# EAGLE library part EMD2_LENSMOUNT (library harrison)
EMD2 Chip
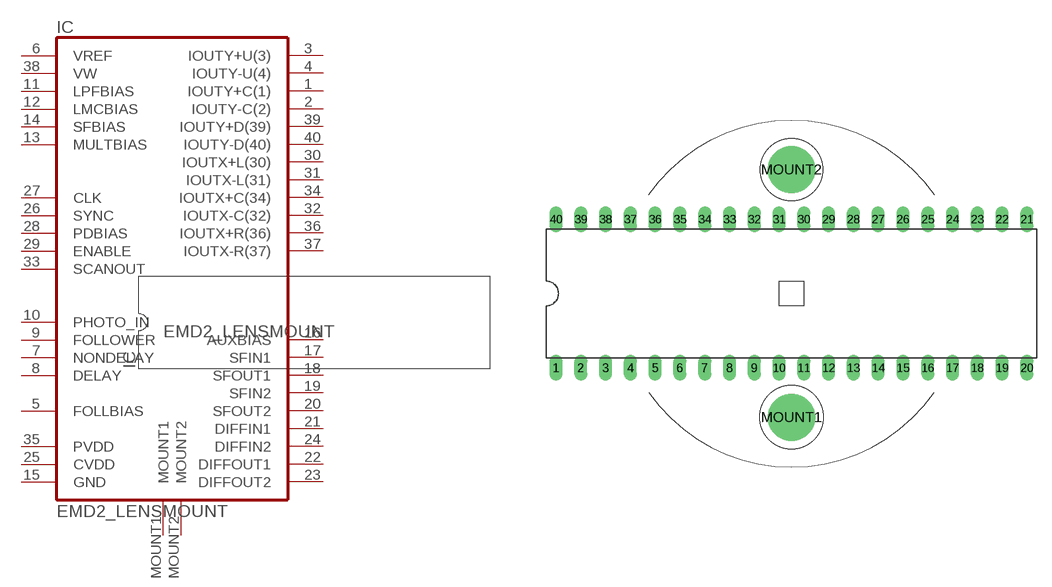
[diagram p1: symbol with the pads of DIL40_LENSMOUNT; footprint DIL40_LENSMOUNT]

Designator prefix IC

## EMD2_LENSMOUNT  [DIL40_LENSMOUNT]
1  IOUTY+C(1)  pas
2  IOUTY-C(2)  pas
3  IOUTY+U(3)  pas
4  IOUTY-U(4)  pas
5  FOLLBIAS  in
6  VREF  pas
7  NONDELAY  out
8  DELAY  out
9  FOLLOWER  out
10  PHOTO_IN  in
11  LPFBIAS  pas
12  LMCBIAS  pas
13  MULTBIAS  pas
14  SFBIAS  pas
15  GND  pwr
16  AUXBIAS  in
17  SFIN1  in
18  SFOUT1  out
19  SFIN2  in
20  SFOUT2  out
21  DIFFIN1  in
22  DIFFOUT1  pas
23  DIFFOUT2  pas
24  DIFFIN2  in
25  CVDD  pwr
26  SYNC  out
27  CLK  in
28  PDBIAS  in
29  ENABLE  in
30  IOUTX+L(30)  pas
31  IOUTX-L(31)  pas
32  IOUTX-C(32)  pas
33  SCANOUT  out
34  IOUTX+C(34)  pas
35  PVDD  pwr
36  IOUTX+R(36)  pas
37  IOUTX-R(37)  pas
38  VW  pas
39  IOUTY+D(39)  pas
40  IOUTY-D(40)  pas
MOUNT1  MOUNT1  pas
MOUNT2  MOUNT2  pas

## Footprint DIL40_LENSMOUNT (pad centres in mm)
drill 0.813 long: 1 -24.13,-7.62; 2 -21.59,-7.62; 3 -19.05,-7.62; 4 -16.51,-7.62; 5 -13.97,-7.62; 6 -11.43,-7.62; 7 -8.89,-7.62; 8 -6.35,-7.62; 9 -3.81,-7.62; 10 -1.27,-7.62; 11 1.27,-7.62; 12 3.81,-7.62; 13 6.35,-7.62; 14 8.89,-7.62; 15 11.43,-7.62; 16 13.97,-7.62; 17 16.51,-7.62; 18 19.05,-7.62; 19 21.59,-7.62; 20 24.13,-7.62; 21 24.13,7.62; 22 21.59,7.62; 23 19.05,7.62; 24 16.51,7.62; 25 13.97,7.62; 26 11.43,7.62; 27 8.89,7.62; 28 6.35,7.62; 29 3.81,7.62; 30 1.27,7.62; 31 -1.27,7.62; 32 -3.81,7.62; 33 -6.35,7.62; 34 -8.89,7.62; 35 -11.43,7.62; 36 -13.97,7.62; 37 -16.51,7.62; 38 -19.05,7.62; 39 -21.59,7.62; 40 -24.13,7.62
drill 3.81: MOUNT1 0,-12.7; MOUNT2 0,12.7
